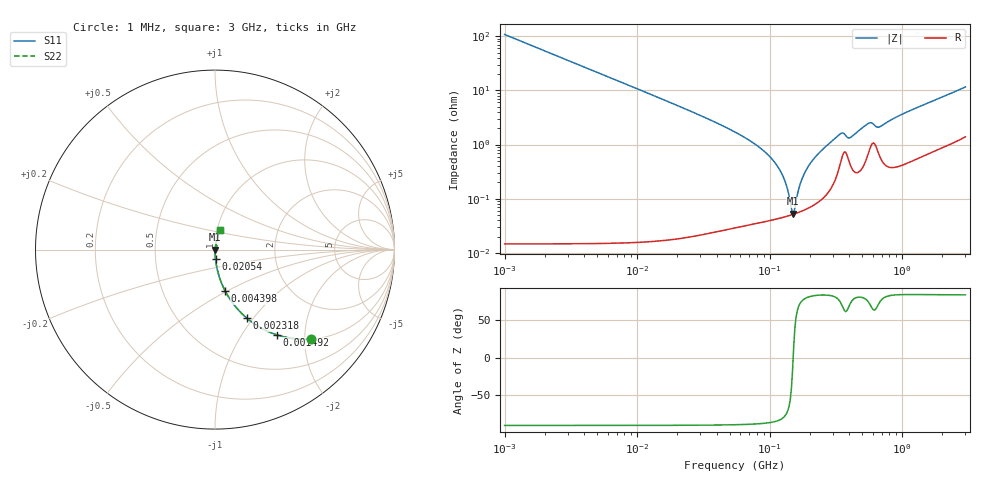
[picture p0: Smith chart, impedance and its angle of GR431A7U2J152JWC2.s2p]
!Murata Part Number: GR431A7U2J152JWC2
!These Parameters are Measured in Series Mode Connection
!Data Generated on Jun 10, 2025
!  o--ll--o
!Port1  Port2
!  o------o
!Operation Temp=25[degC], DC Bias Voltage=0[V]
!Freq. Start=1000[kHz] Stop=3[GHz] 401[Steps]
# Hz S RI R 50
!Freq.(Hz) S11(Real) S11(Imag) S21(Real) S21(Imag) S12(Real) S12(Imag) S22(Real) S22(Imag)
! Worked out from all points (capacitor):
!   401 points, 1 MHz to 3 GHz, reference 50 ohm
!   read as one part in series: C = 1.48 nF near 1.041 MHz
!   lowest |Z| = 53.1 mohm at 149 MHz (marker M1)
!   series resonance near 150.5 MHz, so ESL is about 760 pH
!   S11 on the Smith chart (normalised r, x): 1 MHz: 1.00, -2.16; 1.492 MHz: 1.00, -1.44; 2.318 MHz: 1.00, -0.93; 4.398 MHz: 1.00, -0.49; 20.54 MHz: 1.00, -0.10; 3 GHz: 1.03, +0.23
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1000000  0.5373 -0.4985  0.4627 0.4985  0.4627 0.4985  0.5373 -0.4985
1492300  0.3428 -0.4745  0.6572 0.4745  0.6572 0.4745  0.3428 -0.4745
2317916  0.1778 -0.3822  0.8222 0.3822  0.8222 0.3822  0.1778 -0.3822
3823119  0.0736 -0.2609  0.9264 0.2609  0.9264 0.2609  0.0736 -0.2609
4398124  0.0567 -0.2309  0.9433 0.2309  0.9433 0.2309  0.0567 -0.2309
1.461624e7  0.00546 -0.0726  0.9945 0.0726  0.9945 0.0726  0.00546 -0.0726
2.054061e7  0.00282 -0.0513  0.9972 0.0513  0.9972 0.0513  0.00282 -0.0513
5.477226e7  0.000578 -0.017  0.9994 0.017  0.9994 0.017  0.000578 -0.017
8.338914e7  0.000437 -0.00893  0.9996 0.00893  0.9996 0.00893  0.000437 -0.00893
1.103592e8  0.000437 -0.00451  0.9996 0.00451  0.9996 0.00451  0.000437 -0.00451
1.295243e8  0.000465 -0.00216  0.9995 0.00216  0.9995 0.00216  0.000465 -0.00216
1.49005e8  0.000511 -0.000143  0.9995 0.000143  0.9995 0.000143  0.000511 -0.000143
1.550909e8  0.000528 0.000435  0.9995 -0.000435  0.9995 -0.000435  0.000528 0.000435
1.680187e8  0.00057 0.0016  0.9994 -0.0016  0.9994 -0.0016  0.00057 0.0016
1.784169e8  0.000609 0.00249  0.9994 -0.00249  0.9994 -0.00249  0.000609 0.00249
2.094008e8  0.000755 0.00495  0.9992 -0.00495  0.9992 -0.00495  0.000755 0.00495
3.385367e8  0.00432 0.0148  0.9957 -0.0148  0.9957 -0.0148  0.00432 0.0148
4.0536e8  0.00441 0.0126  0.9956 -0.0126  0.9956 -0.0126  0.00441 0.0126
5.583748e8  0.00759 0.0233  0.9924 -0.0233  0.9924 -0.0233  0.00759 0.0233
6.685918e8  0.00688 0.0197  0.9931 -0.0197  0.9931 -0.0197  0.00688 0.0197
8.005644e8  0.00452 0.0269  0.9955 -0.0269  0.9955 -0.0269  0.00452 0.0269
3e9  0.0262 0.1105  0.9738 -0.1105  0.9738 -0.1105  0.0262 0.1105
